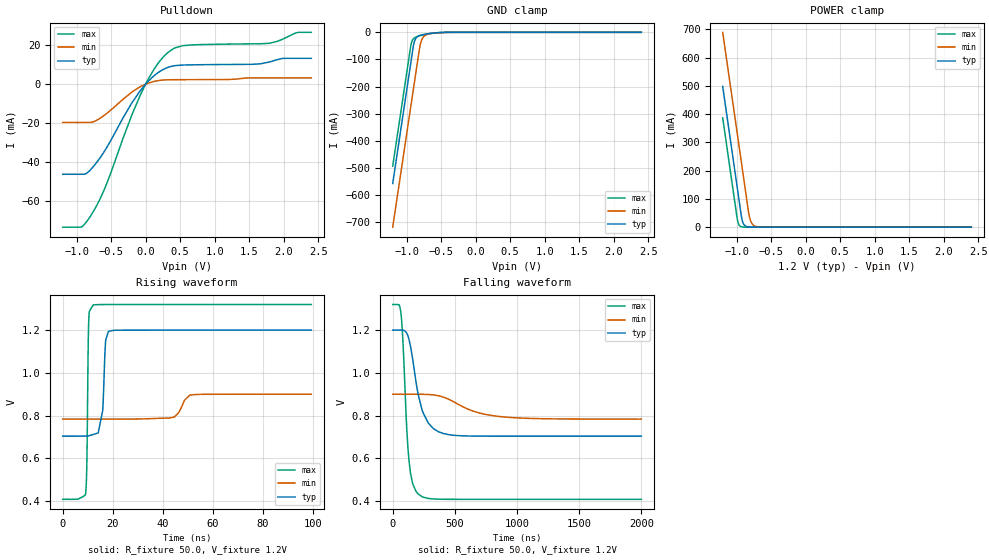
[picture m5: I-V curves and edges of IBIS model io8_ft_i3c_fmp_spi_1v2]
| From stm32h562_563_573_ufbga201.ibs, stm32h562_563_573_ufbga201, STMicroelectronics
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[Model]   io8_ft_i3c_fmp_spi_1v2
Model_type I/O_open_drain
Polarity   Non-Inverting
Enable   Active-Low
| CAP_THRESHOLD on pad IOFT is "UDTCAPC" :
| Rising=20.0% of vddiom   Falling=80.0% of vddiom
| C_comp min and max val. don't necessarily correlate with the min and max pvt
| but are the smallest and greatest pad capacitance found.
| var   typ   min   max
C_comp   3.41530pF  3.39710pF  3.42885pF
|C_comp_pulldown   3.41530pF  3.39710pF  3.42885pF
Vinl = 450.0mV
Vinh = 660.0mV
Vmeas = 600.0mV   | Reference voltage for timing measurements
Cref  = 50.0pF   | Timing specification test load capacitance value
Rref  = 1.0MOhm   | Timing specification test load resistance value
Vref  = 660.0mV   | Timing specification test load voltage
[Model Spec]
| TIME_THRESHOLD on pin ZII2CV11 is "CMOS" :
| Rising=40.0% of vdd   Falling=60.0% of vdd
Vinl 447.80000mV 344.80000mV 489.80000mV
Vinh 733.20000mV 535.20000mV 813.20000mV
| variable   typ   min   max
[Temperature Range] 25.0 125.0 -40.0
| variable   typ   min   max
[Voltage Range] 1.2V 900.0mV 1.32V
| variable   typ   min   max
[POWER Clamp Reference] 1.2V 900.0mV 1.32V
| variable   typ   min   max
[GND Clamp Reference] 0V 0V 0V
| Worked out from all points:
|   slope of the pulldown table from 0 to 0.18 V, typ, clamps not added: 30.6 ohm
|   GND clamp passes 1 mA (typ) near -0.52 V on its own axis
|   POWER clamp passes 1 mA (typ) near -0.84 V on its own axis
|   rising waveform, R_fixture 50.0, V_fixture 1.2V: 20-80 % time 1.27ns typ, 3.39ns min, 533ps max; typ from 0.704 V to 1.2 V
|   falling waveform, R_fixture 50.0, V_fixture 1.2V: 20-80 % time 103ns typ, 287ns min, 47.7ns max; typ from 1.2 V to 0.704 V
[POWER Clamp]
-1.2V     497.8mA    689.2mA    386.5mA
-990mV    140.8mA    332.2mA    29.53mA
-980mV    123.8mA    315.2mA    17.95mA
-960mV    89.81mA    281.2mA    6.634mA
-930mV    38.81mA    230.2mA    1.49mA
-900mV    12.07mA    179.2mA    334.8uA
-870mV    3.756mA    128.2mA    75.22uA
-820mV    536.4uA    44.98mA    6.246uA
-790mV    166.9uA    18.76mA    1.403uA
-750mV    35.18uA    5.846mA    191.8nA
-590mV    70.09nA    55uA       165.5pA
2.4V      0A         0A         0A
[GND Clamp]
-1.2V     -558.2mA   -719mA     -494.1mA
-940mV    -116.2mA   -277mA     -52.06mA
-930mV    -99.19mA   -260mA     -39.94mA
-900mV    -49.1mA    -209mA     -23.76mA
-880mV    -30.14mA   -175mA     -19.6mA
-850mV    -17.82mA   -124mA     -16.09mA
-810mV    -11.73mA   -56.78mA   -12.91mA
-780mV    -9.444mA   -28.21mA   -10.92mA
-740mV    -7.291mA   -13.16mA   -8.574mA
-640mV    -3.573mA   -4.171mA   -3.954mA
-380mV    -61.75uA   -230.3uA   -20.32uA
2.4V      3.863nA    718.4nA    150.6pA
| variable   typ   min   max
[Pullup Reference] 1.2V 900.0mV 1.32V
| variable   typ   min   max
[Pulldown Reference] 0V 0V 0V
[Pulldown]
-1.2V     -46.17mA   -19.61mA   -73.27mA
-930mV    -46.17mA   -19.61mA   -73.18mA
-770mV    -42.8mA    -19.4mA    -66.04mA
-570mV    -32.88mA   -15.17mA   -51.58mA
-200mV    -9.658mA   -4.081mA   -15.89mA
-80mV     -3.488mA   -1.363mA   -5.887mA
120mV     4.232mA    1.386mA    7.501mA
340mV     8.782mA    2.249mA    16.66mA
540mV     9.805mA    2.304mA    19.74mA
1.79V     11.33mA    3.204mA    20.93mA
2.2V      13.23mA    3.204mA    26.48mA
2.4V      13.23mA    3.204mA    26.56mA
[Ramp]
dV/dt_r 297.79693mV/1.03007ns 69.85243mV/3.07748ns 547.1336mV/531.68141ps
dV/dt_f 297.80468mV/100.78484ns 69.85204mV/286.65861ns 547.13918mV/47.66564ns
R_load = 50.0
| Removed startup time: 0s 0s 0s  .
| Removed end time: 99.4ns.
[Rising Waveform]
R_fixture   = 50.0
V_fixture   = 1.2V
V_fixture_min = 900.0mV
V_fixture_max = 1.32V
0s        703.7mV    783.5mV    408.1mV
9.1ns     704mV      783.5mV    429.4mV
9.65ns    704.4mV    783.5mV    575mV
10.15ns   705.1mV    783.5mV    1.092V
10.45ns   705.6mV    783.5mV    1.256V
12.2ns    711.5mV    783.5mV    1.318V
16ns      823.9mV    783.6mV    1.32V
17.1ns    1.139V     783.6mV    1.32V
18.25ns   1.194V     783.6mV    1.32V
99.4ns    1.2V       900mV      1.32V
| Removed startup time: 0s 0s 0s  .
| Removed end time: 1.9994us.
[Falling Waveform]
R_fixture   = 50.0
V_fixture   = 1.2V
V_fixture_min = 900.0mV
V_fixture_max = 1.32V
0s        1.2V       900mV      1.32V
64.75ns   1.2V       900mV      1.286V
79.4ns    1.2V       900mV      1.177V
112.3ns   1.187V     900mV      747.8mV
130.5ns   1.158V     900mV      591.8mV
204.1ns   901mV      900mV      433.5mV
285.7ns   765.6mV    898.8mV    412.3mV
448.9ns   710.9mV    876.9mV    408.2mV
856.9ns   703.7mV    795.9mV    408.1mV
1.999us   703.7mV    783.6mV    408.1mV
